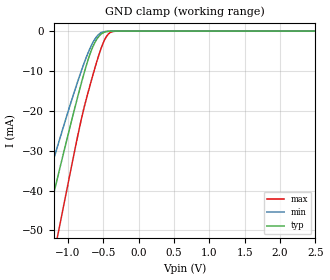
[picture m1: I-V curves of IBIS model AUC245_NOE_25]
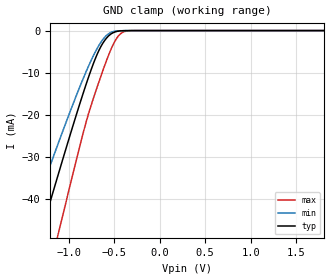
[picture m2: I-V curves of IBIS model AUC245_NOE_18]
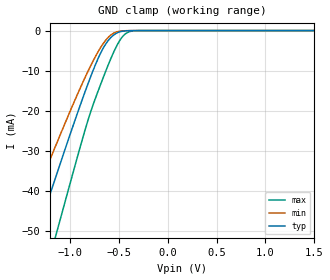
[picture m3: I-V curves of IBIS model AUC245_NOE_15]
| TEXAS INSTRUMENTS INCORPORATED
| Standard Linear and Logic Group
| IBIS Model of SN74AUC245
| Octal Bus Transceiver with 3-State Outputs
| This file contains package information for the following:
|  QFN 20-pin (RGY) package as [Component] AUC245_RGY
|  VFBGA 20-pin (GQN) package as [Component] AUC245_GQN
|  VFBGA 20-pin (ZQN) package as [Component] AUC245_ZQN
| This device can be powered at the following Vccs:
|  2.5 volt Vcc
|  1.8 volt Vcc
|  1.5 volt Vcc
|  1.2 volt Vcc
|  0.8 volt Vcc
| This file provides unique models under the [Model Selector] for each Vcc.
| For operation at a specific Vcc, select the appropriate model after each
| [Model Selector] keyword.
[IBIS Ver]   3.2
[Comment char]  |_char
[File Name]   sn74auc245.ibs
[File Rev]   1.3 | x_die
[Date]   July 13, 2005
[Source]   Data created from TI-SPICE simulations at TI-SLL.
[Notes]   The following is an IBIS list for the AUC245.
   Please contact sllibis@ti.com with questions and
   comments concerning SLL IBIS models.
   - FILE REV HISTORY
   - 1.2 GQN package added on 04/30/04
   - 1.3 ZQN package added on 07/13/05
   - Power clamp data deleted as there is no power-clamp diode.
   - The waveforms for the AUC245_IO Pullup, and
   Pulldown are caused by the circuitry that helps reduce
   overshoot and undershoot in transmission lines (EMI).
   These waveforms are normal for this particular design.
   - End point warning due to AC and DC mismatch.
[Disclaimer] Property of Texas Instruments Incorporated.  Unauthorized
   reproduction and/or distribution is strictly prohibited.
   This product is protected under copyright law.
   Created  2002, (C) Copyright  2002, Texas Instruments
   Incorporated, All Rights Reserved
   UNLESS THERE IS A SIGNED, WRITTEN AGREEMENT TO THE
   CONTRARY, TEXAS INSTRUMENTS (TI) IS PROVIDING THE IBIS
   MODELS  AND WITHOUT ANY WARRANTY, EXPRESSED OR
   IMPLIED.  TI assumes no liability for:
   1) the accuracy of the IBIS models provided to your
   company;
   2) the proper functioning of these IBIS Models in your
   design or for any resulting applications; or
   3) infringement of patents, copyrights or intellectual
   property rights resulting from your use of these IBIS
   models.
   TI provides IBIS Models as a service to our customers.
   You and your company shall not distribute, sell or give
   these models to anyone else without prior written
   permission from TI.
   TI reserves the right to make changes to our products or
   to discontinue any semiconductor product or service
   without notice, and advises our customers to obtain the
   latest version of relevant information to verify, before
   placing orders, that the information being relied on is
   current.
   Please be aware that your receipt and use of the IBIS
   information provided shall serve as acceptance of these
   terms and conditions.  If you do not accept these terms,
   you should return or destroy the IBIS models and any
   other accompanying information immediately.
| Component AUC245_RGY 20-pin QFN
[Component]   AUC245_RGY
[Manufacturer]   Texas Instruments, Inc.
[Package]
|   typ   min   max
R_pkg   0.046   0.035   0.058
L_pkg   1.131nH   0.880nH   1.396nH
C_pkg   0.165pF   0.142pF   0.175pF
[Pin]   signal_name   model_name   R_pin   L_pin   C_pin
1   DIR   AUC245_DIR   0.053   1.289nH   0.142pF
2   A1   AUC245_IO   0.058   1.386nH   0.172pF
3   A2   AUC245_IO   0.046   1.111nH   0.173pF
4   A3   AUC245_IO   0.039   0.965nH   0.161pF
5   A4   AUC245_IO   0.035   0.881nH   0.165pF
6   A5   AUC245_IO   0.035   0.880nH   0.165pF
7   A6   AUC245_IO   0.039   0.961nH   0.161pF
8   A7   AUC245_IO   0.045   1.105nH   0.172pF
9   A8   AUC245_IO   0.058   1.386nH   0.172pF
10   GND   GND   0.056   1.352nH   0.159pF
11   B8   AUC245_IO   0.053   1.287nH   0.155pF
12   B7   AUC245_IO   0.058   1.396nH   0.172pF
13   B6   AUC245_IO   0.047   1.129nH   0.175pF
14   B5   AUC245_IO   0.040   0.976nH   0.164pF
15   B4   AUC245_IO   0.035   0.884nH   0.169pF
16   B3   AUC245_IO   0.035   0.881nH   0.168pF
17   B2   AUC245_IO   0.039   0.967nH   0.162pF
18   B1   AUC245_IO   0.046   1.118nH   0.174pF
19   NOE   AUC245_NOE   0.058   1.396nH   0.175pF
20   VCC   POWER   0.052   1.276nH   0.144pF
| Component AUC245_GQN 20-pin VFBGA
[Component]   AUC245_GQN
[Manufacturer] Texas Instruments, Inc.
[Package]
|   typ   min   max
R_pkg   4.300e-02   3.300e-02   6.100e-02
L_pkg   1.317e-09   8.960e-10   2.088e-09
C_pkg   1.130e-13   6.400e-14   1.900e-13
[Pin]   signal_name   model_name   R_pin   L_pin   C_pin
A2   DIR   AUC245_DIR   3.800e-02   1.199e-09   1.210e-13
A1   A1   AUC245_IO   4.000e-02   1.067e-09   1.020e-13
B3   A2   AUC245_IO   6.100e-02   1.999e-09   1.900e-13
B1   A3   AUC245_IO   3.300e-02   9.630e-10   7.100e-14
C2   A4   AUC245_IO   4.900e-02   1.523e-09   1.230e-13
C1   A5   AUC245_IO   3.300e-02   8.960e-10   6.400e-14
D3   A6   AUC245_IO   6.100e-02   1.899e-09   1.640e-13
D1   A7   AUC245_IO   3.300e-02   8.980e-10   6.700e-14
E2   A3   AUC245_IO   4.900e-02   1.514e-09   1.280e-13
E1   GND   GND   3.600e-02   1.006e-09   9.400e-14
E3   B8   AUC245_IO   4.900e-02   1.683e-09   1.460e-13
E4   B7   AUC245_IO   3.300e-02   1.121e-09   8.900e-14
D2   B6   AUC245_IO   6.100e-02   2.088e-09   1.730e-13
D4   B5   AUC245_IO   3.300e-02   1.027e-09   7.100e-14
C3   B4   AUC245_IO   4.900e-02   1.558e-09   1.240e-13
C4   B3   AUC245_IO   3.300e-02   9.280e-10   6.700e-14
B2   B2   AUC245_IO   6.100e-02   1.921e-09   1.770e-13
B4   B1   AUC245_IO   3.300e-02   9.010e-10   7.700e-14
A4   NOE   AUC245_NOE   3.700e-02   9.900e-10   9.800e-14
A3   VCC   POWER   3.500e-02   1.168e-09   1.190e-13
| Component AUC245_ZQN 20-pin VFBGA
[Component]   AUC245_ZQN
[Manufacturer] Texas Instruments, Inc.
[Package]
|   typ   min   max
R_pkg   4.300e-02   3.300e-02   6.100e-02
L_pkg   1.317e-09   8.960e-10   2.088e-09
C_pkg   1.130e-13   6.400e-14   1.900e-13
[Pin]   signal_name   model_name   R_pin   L_pin   C_pin
A2   DIR   AUC245_DIR   3.800e-02   1.199e-09   1.210e-13
A1   A1   AUC245_IO   4.000e-02   1.067e-09   1.020e-13
B3   A2   AUC245_IO   6.100e-02   1.999e-09   1.900e-13
B1   A3   AUC245_IO   3.300e-02   9.630e-10   7.100e-14
C2   A4   AUC245_IO   4.900e-02   1.523e-09   1.230e-13
C1   A5   AUC245_IO   3.300e-02   8.960e-10   6.400e-14
D3   A6   AUC245_IO   6.100e-02   1.899e-09   1.640e-13
D1   A7   AUC245_IO   3.300e-02   8.980e-10   6.700e-14
E2   A3   AUC245_IO   4.900e-02   1.514e-09   1.280e-13
E1   GND   GND   3.600e-02   1.006e-09   9.400e-14
E3   B8   AUC245_IO   4.900e-02   1.683e-09   1.460e-13
E4   B7   AUC245_IO   3.300e-02   1.121e-09   8.900e-14
D2   B6   AUC245_IO   6.100e-02   2.088e-09   1.730e-13
D4   B5   AUC245_IO   3.300e-02   1.027e-09   7.100e-14
C3   B4   AUC245_IO   4.900e-02   1.558e-09   1.240e-13
C4   B3   AUC245_IO   3.300e-02   9.280e-10   6.700e-14
B2   B2   AUC245_IO   6.100e-02   1.921e-09   1.770e-13
B4   B1   AUC245_IO   3.300e-02   9.010e-10   7.700e-14
A4   NOE   AUC245_NOE   3.700e-02   9.900e-10   9.800e-14
A3   VCC   POWER   3.500e-02   1.168e-09   1.190e-13
| Model AUC245_NOE
[Model Selector]   AUC245_NOE
AUC245_NOE_25   2.5 volt Vcc
AUC245_NOE_18   1.8 volt Vcc
AUC245_NOE_15   1.5 volt Vcc
AUC245_NOE_12   1.2 volt Vcc
AUC245_NOE_08   0.8 volt Vcc
| Model AUC245_DIR
[Model Selector]   AUC245_DIR
AUC245_DIR_25   2.5 volt Vcc
AUC245_DIR_18   1.8 volt Vcc
AUC245_DIR_15   1.5 volt Vcc
AUC245_DIR_12   1.2 volt Vcc
AUC245_DIR_08   0.8 volt Vcc
| Model AUC245_IO
[Model Selector]   AUC245_IO
AUC245_IO_25   2.5 volt Vcc
AUC245_IO_18   1.8 volt Vcc
AUC245_IO_15   1.5 volt Vcc
AUC245_IO_12   1.2 volt Vcc
AUC245_IO_08   0.8 volt Vcc
| Models and submodels in the file (15): AUC245_NOE_25 (Input), AUC245_NOE_18 (Input), AUC245_NOE_15 (Input), AUC245_NOE_12 (Input), AUC245_NOE_08 (Input), AUC245_DIR_25 (Input), AUC245_DIR_18 (Input), AUC245_DIR_15 (Input), AUC245_DIR_12 (Input), AUC245_DIR_08 (Input), AUC245_IO_25 (3-state), AUC245_IO_18 (3-state), AUC245_IO_15 (3-state), AUC245_IO_12 (3-state), AUC245_IO_08 (3-state)
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[Model]   AUC245_NOE_25
Model_type  Input
Vinl=0.7
Vinh=1.7
| variable   typ   min   max
C_comp   2.38pF   1.92pF   2.79pF
[Temperature Range]   40   100   -40
| Ambient temperature   25   85   -40
[Voltage range]   2.5   2.3   2.7
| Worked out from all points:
|   GND clamp passes 1 mA (typ) near -0.55 V on its own axis
[GND Clamp]
| AUC245_NOE_25
|   Voltage   I(typ)   I(min)   I(max)
-3.6V     -222.3mA   -186.1mA   -267.5mA
-1.49V    -62.29mA   -49.79mA   -82.1mA
-1.35V    -51.8mA    -41.14mA   -69.63mA
-1.305V   -48.45mA   -38.39mA   -65.61mA
-1.17V    -38.46mA   -30.25mA   -53.55mA
-1.12V    -34.79mA   -27.28mA   -49.08mA
-735mV    -8.324mA   -6.331mA   -16.67mA
-635mV    -3.426mA   -2.471mA   -10.25mA
-525mV    -682.5uA   -360.4uA   -4.021mA
-430mV    -73.19uA   -34.73uA   -776.9uA
-325mV    -3.339uA   -2.006uA   -30.74uA
2.5V      313.9pA    400.9pA    470.4pA
[Model]   AUC245_NOE_18
Model_type  Input
Vinl=0.5775
Vinh=1.2675
| variable   typ   min   max
C_comp   2.45pF   1.99pF   2.87pF
[Temperature Range]   40   100   -40
| Ambient temperature   25   85   -40
[Voltage range]   1.8   1.65   1.95
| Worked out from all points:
|   GND clamp passes 1 mA (typ) near -0.55 V on its own axis
[GND Clamp]
| AUC245_NOE_18
|   Voltage   I(typ)   I(min)   I(max)
-3.6V     -222.3mA   -186.1mA   -267.5mA
-1.475V   -61.16mA   -48.85mA   -80.77mA
-1.43V    -57.79mA   -46.07mA   -76.76mA
-1.295V   -47.7mA    -37.79mA   -64.71mA
-1.145V   -36.62mA   -28.76mA   -51.31mA
-1.095V   -32.97mA   -25.81mA   -46.85mA
-830mV    -14.31mA   -10.96mA   -23.64mA
-685mV    -5.607mA   -4.224mA   -13.41mA
-560mV    -1.272mA   -753.7uA   -5.827mA
-485mV    -290.6uA   -140.2uA   -2.305mA
-420mV    -55.81uA   -26.72uA   -608.5uA
1.8V      203.2pA    297.2pA    235.5pA
[Model]   AUC245_NOE_15
Model_type  Input
Vinl=0.49
Vinh=1.04
| variable   typ   min   max
C_comp   2.48pF   2.04pF   2.85pF
[Temperature Range]   40   100   -40
| Ambient temperature   25   85   -40
[Voltage range]   1.5   1.4   1.6
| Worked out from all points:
|   GND clamp passes 1 mA (typ) near -0.55 V on its own axis
[GND Clamp]
| AUC245_NOE_15
|   Voltage   I(typ)   I(min)   I(max)
-3.6V     -222.3mA   -186.1mA   -267.5mA
-1.505V   -63.42mA   -50.72mA   -83.44mA
-1.325V   -49.94mA   -39.61mA   -67.39mA
-1.17V    -38.46mA   -30.25mA   -53.55mA
-1.12V    -34.79mA   -27.28mA   -49.08mA
-840mV    -14.98mA   -11.48mA   -24.46mA
-695mV    -6.114mA   -4.621mA   -14.06mA
-570mV    -1.487mA   -911.6uA   -6.381mA
-495mV    -364.6uA   -178.8uA   -2.692mA
-430mV    -73.19uA   -34.73uA   -776.9uA
-280mV    -781.4nA   -556.3nA   -5.358uA
1.5V      165.9pA    258.5pA    172.1pA
